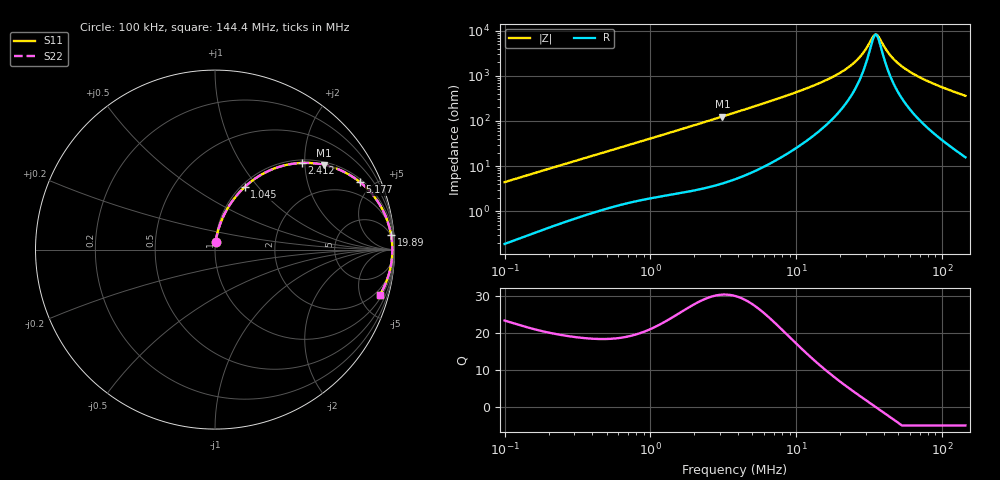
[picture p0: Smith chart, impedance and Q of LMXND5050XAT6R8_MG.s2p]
! LMXND5050XAT6R8_MG  S-PARAMETER MODEL  ( General Type )
! Model Generated by TAIYO YUDEN Corporation (https://www.yuden.co.jp/en/)
! Version 1.0
! TAIYO YUDEN Control No. 191023NI43SB-FBB
! Copyright(c) 2019 TAIYO YUDEN CO.,LTD. All Rights Reserved.
! Product Description (link to TY-COMPAS)
! https://ds.yuden.co.jp/TYCOMPAS/or/detail?pn=LMXND5050XAT6R8MMG&u=M
! Products Name : Inductors
! Characteristics :
!  Inductance : 6.8 uH , SRF(min) : 22 MHz , DC Resistance(max) : 0.0676 Ohm
!  Rated Current : Saturation :2500 mA , Temp Rise : 2300 mA (40 degC)
!  Case Size : 4.9 x 4.9 / 0.193 x 0.193 [mm/inch] , Thickness : 3.1 / 0.122 [mm/inch]
!  (Conditions: Temperature = 25 degC , DC Bias Current/Voltage = 0A / 0V)
! External Node Assignments :
!  1  o---GGG---o  2
! GND o---------o GND
! Frequency Range : 0.1MHz  -  144.390904MHz  [ 402 STEP ]
# MHz S RI R 50
! Freq[MHz].  S11 Real  S11 Imag  S21 Real  S21 Imag  S12 Real  S12 Imag  S22 Real  S22 Imag
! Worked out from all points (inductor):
!   401 points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, 100 kHz to 144.4 MHz, reference 50 ohm
!   read as one part in series: L = 6.99 uH near 103.7 kHz
!   highest Q = 30.4 at 3.111 MHz (marker M1), where L = 6.4 uH
!   self-resonance near 34.95 MHz
!   S11 on the Smith chart (normalised r, x): 100 kHz: 1.00, +0.09; 1.045 MHz: 1.04, +0.85; 2.412 MHz: 1.07, +1.94; 5.177 MHz: 1.15, +4.21; 19.89 MHz: 4, +23; 144.4 MHz: 1.31, -7.19
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0.1  0.00383 0.0439  0.9962 -0.0439  0.9962 -0.0439  0.00383 0.0439
0.338238  0.0274 0.1388  0.9726 -0.1388  0.9726 -0.1388  0.0274 0.1388
0.639268  0.0768 0.2409  0.9232 -0.2409  0.9232 -0.2409  0.0768 0.2409
1.044604  0.1644 0.348  0.8356 -0.348  0.8356 -0.348  0.1644 0.348
1.144052  0.1882 0.369  0.8118 -0.369  0.8118 -0.369  0.1882 0.369
2.411563  0.4848 0.483  0.5152 -0.483  0.5152 -0.483  0.4848 0.483
3.110875  0.6069 0.4723  0.3931 -0.4723  0.3931 -0.4723  0.6069 0.4723
3.869624  0.703 0.4405  0.297 -0.4405  0.297 -0.4405  0.703 0.4405
5.176669  0.8075 0.3764  0.1925 -0.3764  0.1925 -0.3764  0.8075 0.3764
7.865456  0.905 0.2705  0.095 -0.2705  0.095 -0.2705  0.905 0.2705
12.85266  0.9604 0.1605  0.0396 -0.1605  0.0396 -0.1605  0.9604 0.1605
19.88681  0.9807 0.0831  0.0193 -0.0831  0.0193 -0.0831  0.9807 0.0831
26.60399  0.9864 0.0391  0.0136 -0.0391  0.0136 -0.0391  0.9864 0.0391
29.67153  0.9874 0.0235  0.0126 -0.0235  0.0126 -0.0235  0.9874 0.0235
33.70015  0.9879 0.00561  0.0121 -0.00561  0.0121 -0.00561  0.9879 0.00561
34.94858  0.988 0.000521  0.012 -0.000521  0.012 -0.000521  0.988 0.000521
36.90848  0.9879 -0.00711  0.0121 0.00711  0.0121 0.00711  0.9879 -0.00711
43.47261  0.9871 -0.0302  0.0129 0.0302  0.0129 0.0302  0.9871 -0.0302
52.14399  0.9848 -0.0567  0.0152 0.0567  0.0152 0.0567  0.9848 -0.0567
66.05251  0.9791 -0.0937  0.0209 0.0937  0.0209 0.0937  0.9791 -0.0937
93.31843  0.9629 -0.1557  0.0371 0.1557  0.0371 0.1557  0.9629 -0.1557
144.3909  0.919 -0.2519  0.081 0.2519  0.081 0.2519  0.919 -0.2519
